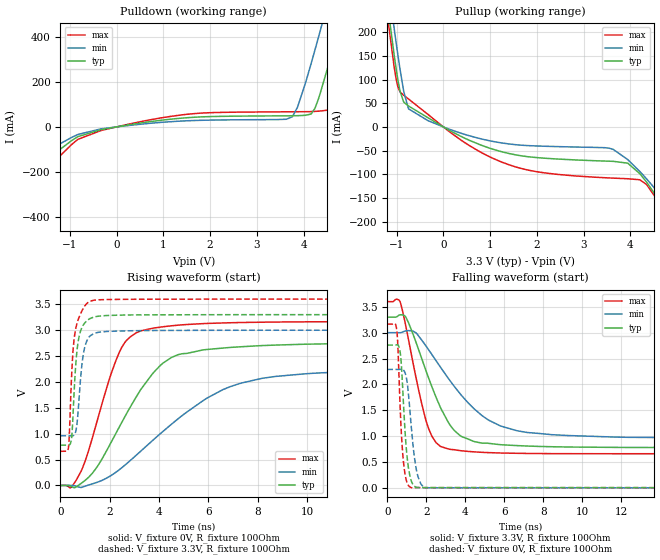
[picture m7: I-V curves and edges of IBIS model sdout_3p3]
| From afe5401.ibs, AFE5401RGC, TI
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|   sdout_3p3 Model
[Model]   sdout_3p3
Model_type   Output
Polarity   Non-Inverting
Vmeas = 1.65
Vref = 0
Cref = 5pF
Rref = 50
|   typ   min   max
|   (nom PVT)   (fast PVT)   (slow PVT)
C_comp   1.593e-12   1.546e-12   1.650e-12
| Where nom  PVT is Nominal Process, 3.3V, 27C
|   Fast PVT is Strong Process,  3.6V, -40C
|   Slow PVT is Weak Process,   3V, 125C
[Voltage Range]   3.3   3   3.6
|Junction Temperature
[Temperature Range]   27   125   -40
[Pullup Reference]   3.3   3   3.6
[Pulldown Reference]   0   0   0
[Power Clamp Reference]   3.3   3   3.6
[GND Clamp Reference]   0   0   0
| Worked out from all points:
|   slope of the pulldown table from 0 to 0.495 V, typ, clamps not added: 29.3 ohm
|   slope of the pullup table from 0 to 0.495 V, typ, clamps not added: 19.3 ohm
|   falling waveform, V_fixture 3.3V, R_fixture 100Ohm: 20-80 % time 1.62ns typ, 2.71ns min, 1.02ns max; typ from 3.3 V to 0.779 V
|   rising waveform, V_fixture 0V, R_fixture 100Ohm: 20-80 % time 2.09ns typ, 3.73ns min, 1.24ns max; typ from 0 V to 2.76 V
|   rising waveform, V_fixture 3.3V, R_fixture 100Ohm: 20-80 % time 223ps typ, 244ps min, 229ps max; typ from 0.779 V to 3.3 V
|   falling waveform, V_fixture 0V, R_fixture 100Ohm: 20-80 % time 280ps typ, 365ps min, 235ps max; typ from 2.76 V to 0 V
[Pulldown]
|   Voltage   I(typ)   I(min)   I(max)
-3.3V     -1.138A    -961.7mA   -1.29A
-2.385V   -573.8mA   -443.7mA   -689.2mA
-2.004V   -357.7mA   -251.6mA   -455.3mA
-1.508V   -147.3mA   -109.6mA   -189.8mA
-823.2mV  -43.01mA   -33.45mA   -54.95mA
3.762V    49.64mA    45.5mA     67.55mA
4.163V    57.72mA    282mA      68.34mA
4.354V    147mA      425mA      70.8mA
4.503V    253.7mA    540.1mA    74.49mA
4.858V    528.5mA    819.1mA    269.4mA
5.188V    793.7mA    1.083A     532mA
6.6V      1.971A     2.245A     1.724A
[Pullup]
|   Voltage   I(typ)   I(min)   I(max)
-3.3V     2.002A     2.025A     2.009A
-1.233V   287mA      343.1mA    261.8mA
-1.057V   154.3mA    210.8mA    129.3mA
-927.3mV  75.19mA    121.2mA    74.16mA
-747mV    44.26mA    38.27mA    59.03mA
-330mV    19.48mA    13.28mA    26.43mA
1.405V    -56.19mA   -36.01mA   -80.04mA
3.627V    -72.67mA   -47.28mA   -108.2mA
3.943V    -76.61mA   -68.97mA   -109.5mA
4.346V    -116.6mA   -109.7mA   -121.7mA
4.973V    -225.2mA   -254.2mA   -225.1mA
6.6V      -1.212A    -1.184A    -1.197A
[Ramp]
R_load = 100
|   typ   min   max
dV/dt_r   1.65611/2.09253e-09   1.37317/3.71838e-09   1.89978/1.23469e-09
dV/dt_f   1.51265/1.61654e-09   1.22449/2.71045e-09   1.7642/1.01865e-09
[Falling Waveform]
V_fixture = 3.3V
V_fixture_min = 3V
V_fixture_max = 3.6V
R_fixture = 100Ohm
|   Time   V(typ)   V(min)   V(max)
0s        3.3V       3V         3.6V
670ps     3.346V     3V         3.581V
1.06ns    3.216V     3.04V      2.917V
1.76ns    2.505V     2.86V      1.637V
2.27ns    1.972V     2.587V     1.013V
3.11ns    1.281V     2.128V     755.1mV
3.81ns    992.4mV    1.787V     716.3mV
6.67ns    816.7mV    1.103V     668mV
11.75ns   782.2mV    981mV      659.6mV
75ns      778.9mV    959.2mV    659.7mV
[Rising Waveform]
V_fixture = 0V
V_fixture_min = 0V
V_fixture_max = 0V
R_fixture = 100Ohm
|   Time   V(typ)   V(min)   V(max)
0s        1.791nV    92.44nV    914.2pV
420ps     -14.58mV   991.3uV    -42.56mV
860ps     46.84mV    -36.9mV    299mV
2.04ns    820.9mV    187.9mV    2.138V
2.61ns    1.327V     391.2mV    2.762V
3.71ns    2.145V     857.7mV    3.034V
4.77ns    2.526V     1.288V     3.097V
7.33ns    2.68V      1.978V     3.148V
11.91ns   2.744V     2.209V     3.165V
75ns      2.76V      2.289V     3.166V
[Rising Waveform]
V_fixture = 3.3V
V_fixture_min = 3V
V_fixture_max = 3.6V
R_fixture = 100Ohm
|   Time   V(typ)   V(min)   V(max)
0s        778.9mV    959.2mV    659.7mV
330ps     779.4mV    959.4mV    754mV
460ps     959.1mV    957.8mV    2.198V
520ps     1.465V     963mV      2.662V
620ps     2.33V      1.045V     3.033V
760ps     2.885V     1.718V     3.253V
870ps     3.052V     2.331V     3.372V
970ps     3.131V     2.641V     3.457V
1.42ns    3.261V     2.946V     3.583V
75ns      3.3V       3V         3.6V
[Falling Waveform]
V_fixture = 0V
V_fixture_min = 0V
V_fixture_max = 0V
R_fixture = 100Ohm
|   Time   V(typ)   V(min)   V(max)
0s        2.76V      2.289V     3.166V
470ps     2.764V     2.288V     3.091V
650ps     2.645V     2.29V      1.637V
760ps     2.135V     2.29V      818.9mV
900ps     1.155V     2.232V     286.3mV
1.06ns    452.6mV    1.906V     61.31mV
1.26ns    107.8mV    1.06V      2.017mV
1.53ns    6.712mV    280.8mV    5.532mV
1.99ns    5.474mV    993.5uV    3.605mV
75ns      438.8pV    91.19nV    -1.859nV
